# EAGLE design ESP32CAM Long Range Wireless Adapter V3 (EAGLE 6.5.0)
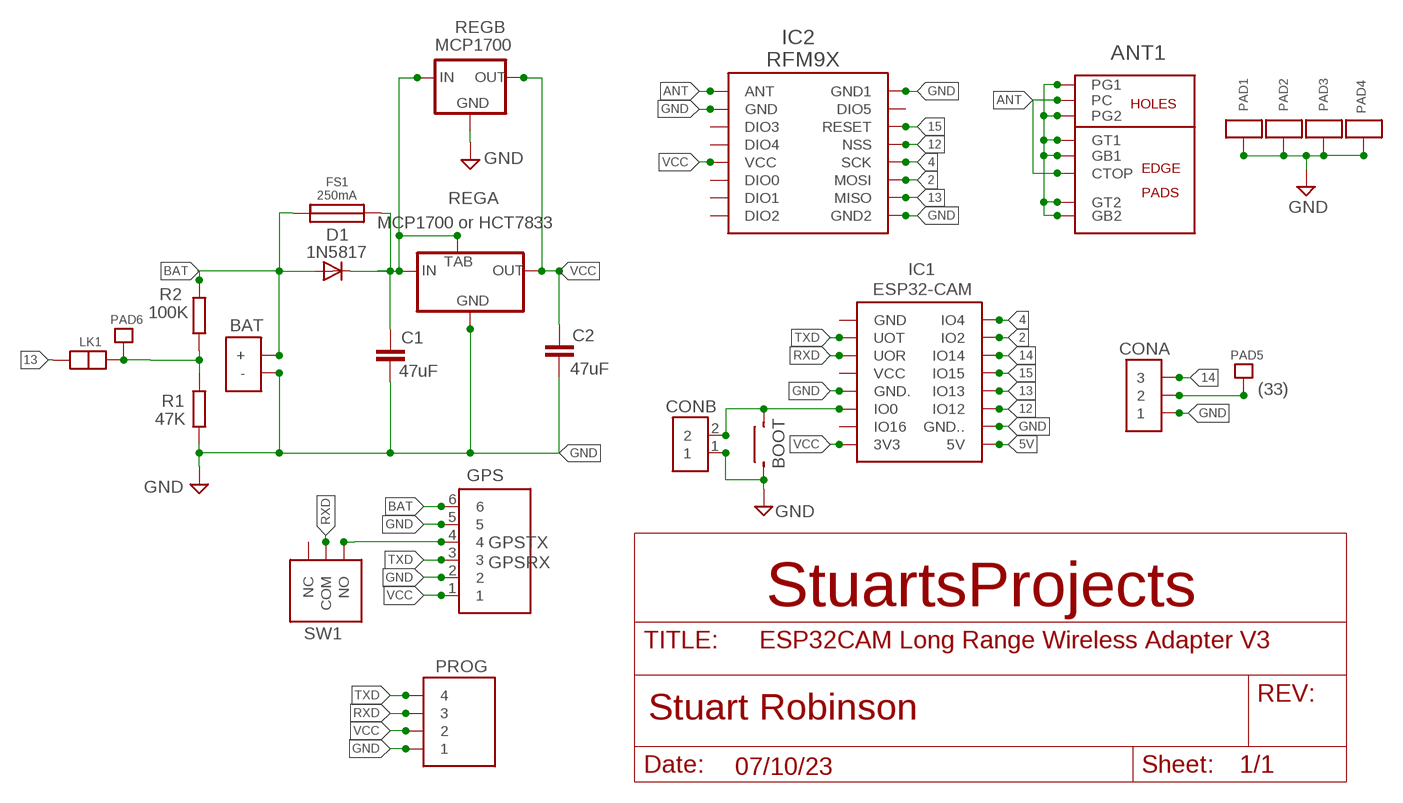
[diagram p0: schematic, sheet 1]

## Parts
ANT1  CUSTOMSMA  [CUSTOMSMA]
BAT  BATPADS2  [BATPADS]
BOOT  SMALLSMTSWITCH  [SMALLSMTSWITCH]
C1  47uF  C-EUC1206  [C1206]
C2  47uF  C-EUC1206  [C1206]
CONA  3X1  [3X1]
CONB  2X1  [2X1]
D1  1N5817  DIODE-DO41-7.6  [DO41-7.6]
FS1  250mA  SMALL_POLYFUSE  [SMALL_POLYFUSE]
GPS  6X1  [6X1]
IC1  ESP32-CAM  [ESP32-CAM]
IC2  RFM9X  RFM98_PIH  [RFM98_PIH]
LK1  2PADLINKLARGE  [2PADLINKLARGE]
PAD1  ANTPAD2  [ANTPAD2]
PAD2  ANTPAD2  [ANTPAD2]
PAD3  ANTPAD2  [ANTPAD2]
PAD4  ANTPAD2  [ANTPAD2]
PAD5  SINGLEPAD  [SINGLEPAD]
PAD6  SINGLEPAD  [SINGLEPAD]
PROG  4X1  [4X1]
R1  47K  125MWRESISTORSTANDARD  [125MWRESISTOR]
R2  100K  125MWRESISTORSTANDARD  [125MWRESISTOR]
REGA  MCP1700 or HCT7833  MCP1700SOT89  [MCP1700SOT89]
REGB  MCP1700  [TO92REGB]
SW1  SMALL_PCB_SLIDE_DEFAULT  [SMALL_PCB_SLIDE]

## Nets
2: IC1.IO2 IC2.MOSI
4: IC1.IO4 IC2.SCK
5V [POWER]: C1.1 D1.C FS1.P$2 IC1.5V REGA.2(IN) REGA.4(TAB) REGB.IN
12: IC1.IO12 IC2.NSS
13: IC1.IO13 IC2.MISO LK1.P$1
14: CONA.3 IC1.IO14
15: IC1.IO15 IC2.RESET
ANT: ANT1.CTOP ANT1.PC IC2.ANT
BAT [POWER]: BAT.BAT+(+) D1.A FS1.P$1 GPS.6 R2.P$1
GND [POWER]: ANT1.G1 ANT1.G2 ANT1.GB1 ANT1.GB2 ANT1.GT1 ANT1.GT2 BAT.BAT-V(-) BOOT.P$3 C1.2 C2.2 CONA.1 CONB.1 GPS.2 GPS.5 IC1.GND. IC1.GND.. IC2.GND IC2.GND1 IC2.GND2 PAD1.P$1 PAD2.P$1 PAD3.P$1 PAD4.P$1 PROG.1 R1.P$2 REGA.1(GND) REGB.GND
N$1: BOOT.P$4 CONB.2 IC1.IO0
N$2: CONA.2 PAD5.P$1
N$3: GPS.4 SW1.NO
PAD6: LK1.P$2 PAD6.P$1 R1.P$1 R2.P$2
RXD: IC1.UOR PROG.3 SW1.COM
TXD: GPS.3 IC1.UOT PROG.4
VCC [POWER]: C2.1 GPS.1 IC1.3V3 IC2.VCC PROG.2 REGA.3(OUT) REGB.OUT
Unconnected: IC1.GND IC1.IO16 IC1.VCC IC2.DIO0 IC2.DIO1 IC2.DIO2 IC2.DIO3 IC2.DIO4 IC2.DIO5 SW1.NC

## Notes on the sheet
- (33)
- GPSTX
- GPSRX
- StuartsProjects
- 07/10/23

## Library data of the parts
ANT1 = con-coax:CUSTOMSMA
BAT = LMA2:BATPADS2
BOOT = LMA2:SMALLSMTSWITCH
C1 C2 = resistor:C-EU: CAPACITOR, European symbol
CONA = My_Pin_Headers:3X1
CONB = My_Pin_Headers:2X1
D1 = diode:DIODE-: DIODE
FS1 = LMA2:SMALL_POLYFUSE
GPS = My_Pin_Headers:6X1
IC1 = esp32:ESP32-CAM
IC2 = LMA2:RFM98_PIH
LK1 = LMA2:2PADLINKLARGE
PAD1-PAD4 = LMA2:ANTPAD2
PAD5 PAD6 = LMA2:SINGLEPAD
PROG = My_Pin_Headers:4X1
R1 R2 = LMA2:125MWRESISTOR
REGA = LMA2:MCP1700SOT89
REGB = LMA2:MCP1700
SW1 = switch-tact:SMALL_PCB_SLIDE

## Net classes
0 default: width 0.254 mm
1 POWER: width 0.762 mm
2 VDD: width 0.762 mm
3 gpspower: width 0.762 mm

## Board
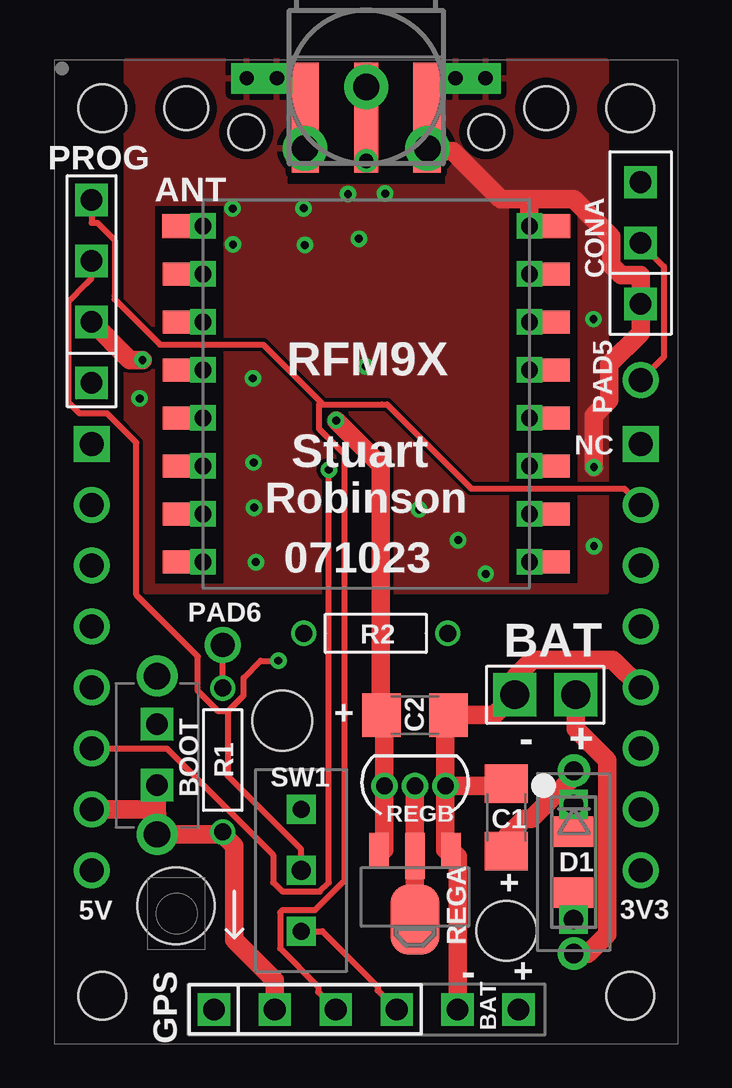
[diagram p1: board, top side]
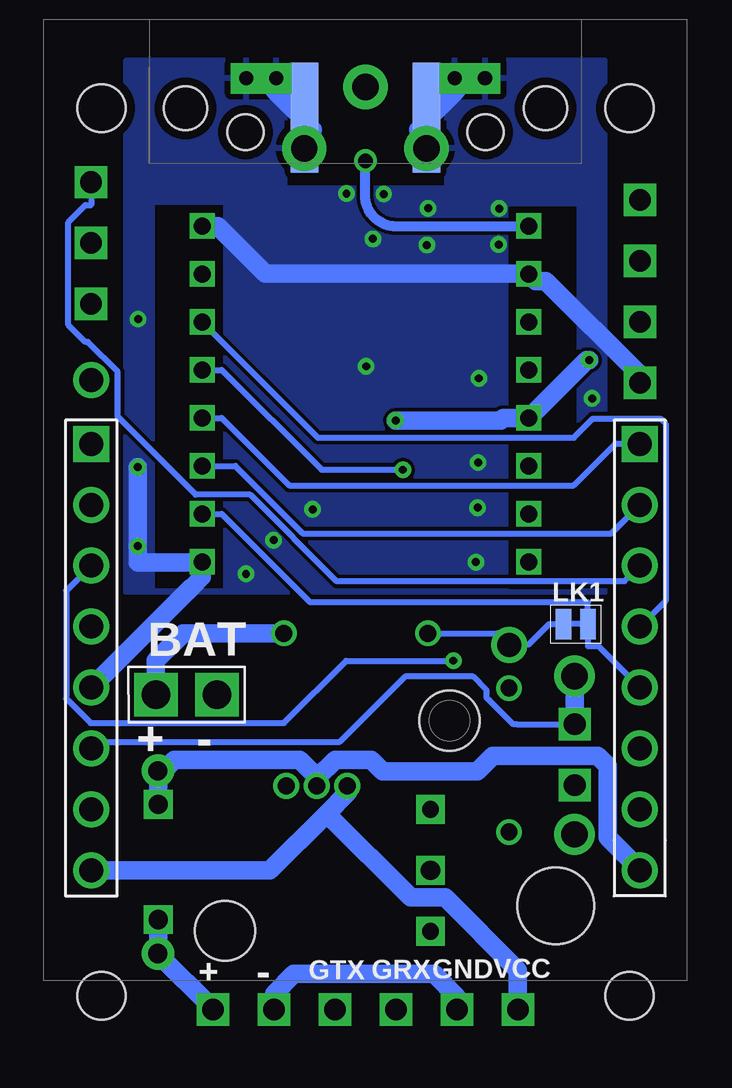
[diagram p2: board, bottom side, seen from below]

No outline drawn. Coordinates in mm, seen from the top.
Copper layers (1*16): Top 0.0356mm / dielectric 1.5011mm / Bottom 0.0356mm
Design rules "LaenPCBOrder *": minimum track width 6mil, minimum drill 13mil, track to track 6mil, track to pad 6mil, pad to pad 6mil, via to via 6mil, smd to smd 6mil, copper to edge 15mil, drill to drill 6mil, minimum pad ring 7mil, minimum via ring 7mil, stop-mask expansion 3mil, vias tented up to drill 1000mil, thermal gap 10mil
Holes 3.2 mm at 5.07,5.75
Holes 1.5 mm at 8,38 18,38
Holes 2.5 mm at 9.5,13.47 18.85,4.71
Holes 2 mm at 2,2 24,2 2,39 24,39
Holes 1.8 mm at 5.5,39 20.5,39
tRestrict: area 0,0 to 26.4,0.5; area 9.7,35.9 to 16.3,41; area 4.2,19.2 to 7,34.9; area 19,19.2 to 21.8,34.9
bRestrict: area 0,0 to 26.1,0.5; area 9.7,35.8 to 16.2,41; area 4.2,19 to 7,34.9; area 18.9,19 to 21.8,35

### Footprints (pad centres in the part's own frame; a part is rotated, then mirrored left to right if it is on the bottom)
CUSTOMSMA = smd 4.572 x 1.016: CTOP -1.27,0 | drill 1.1 pad 1.85: G1 -2.55,2.55; G2 -2.55,-2.55; PC 0,0 | smd 4.572 x 1.143 bottom: GB1 -1.27,2.54; GB2 -1.27,-2.54 | smd 4.572 x 1.143: GT1 -1.27,2.54; GT2 -1.27,-2.54
BATPADS = drill 1.2 pad 1.778 square: BAT+ 0,-1.27; BAT-V 0,1.27
SMALLSMTSWITCH = drill 1.1 pad 1.7: P$3 -3.3,0; P$4 3.3,0
C1206 = smd 1.6 x 1.8: 1 -1.4,0; 2 1.4,0
3X1 = drill 0.9 square: 1 -2.54,0; 2 0,0; 3 2.54,0
2X1 = drill 0.9 square: 1 -1.27,0; 2 1.27,0
DO41-7.6 = drill 0.8 pad 1.35: A 3.81,0; C -3.81,0
SMALL_POLYFUSE = drill 0.8 square: P$1 -2.4,0; P$2 2.4,0 | smd 1.27 x 1.635: P$3 -1.27,0; P$4 1.27,0
6X1 = drill 0.9 square: 1 -6.35,0; 2 -3.81,0; 3 -1.27,0; 4 1.27,0; 5 3.81,0; 6 6.35,0
ESP32-CAM = drill 1: 3V3 -11.43,3.81; 5V 11.43,3.81; GND. -11.43,11.43; GND.. 11.43,6.35; IO0 -11.43,8.89; IO2 11.43,19.05; IO12 11.43,8.89; IO13 11.43,11.43; IO14 11.43,16.51; IO15 11.43,13.97; IO16 -11.43,6.35; UOR -11.43,16.51; UOT -11.43,19.05; VCC -11.43,13.97 | drill 1 square: GND -11.43,21.59; IO4 11.43,21.59
RFM98_PIH = drill 0.7 pad 0.965 square: ANT -6.8,7.5; DIO0 -6.8,-2.5; DIO1 -6.8,-4.5; DIO2 -6.8,-6.5; DIO3 -6.8,3.5; DIO4 -6.8,1.5; DIO5 6.8,5.5; GND -6.8,5.5; GND2 6.8,-6.5; MISO 6.8,-4.5; MOSI 6.8,-2.5; NSS 6.8,1.5; RESET 6.8,3.5; SCK 6.8,-0.5; VCC -6.8,-0.5 | drill 0.7 pad 1.016 square: GND1 6.8,7.5 | smd 2.2 x 1: P$2 -7.4,7.5; P$6 7.4,7.5 | smd 2.159 x 0.965: P$4 -7.4,5.5; P$5 -7.4,1.5; P$7 7.4,5.5; P$9 -7.4,3.5; P$10 -7.4,-0.5; P$11 -7.4,-2.5; P$12 -7.4,-4.5; P$13 -7.4,-6.5; P$14 7.4,-6.5; P$15 7.4,-4.5; P$16 7.4,-2.5; P$17 7.4,-0.5; P$18 7.4,1.5; P$19 7.4,3.5
2PADLINKLARGE = smd 1.27 x 0.66: P$1 0,0.46; P$2 0,-0.56
ANTPAD2 = drill 0.6 pad 1.27 square: P$1 0,0
SINGLEPAD = drill 1: P$1 0,0
4X1 = drill 0.9 square: 1 -3.81,0; 2 -1.27,0; 3 1.27,0; 4 3.81,0
125MWRESISTOR = drill 0.7: P$1 -3,0; P$2 3,0
MCP1700SOT89 = smd 0.8 x 1.4: 1 -1.499,-1.981; 3 1.499,-1.981 | smd 0.8 x 1.9: 2 0,-1.727 | smd 2.032 x 2.921: 4 0,0.94
TO92REGB = drill 0.7 pad 1.1: GND -1.27,-1.2; IN 0,-1.2; OUT 1.27,-1.2
SMALL_PCB_SLIDE = drill 0.8 pad 1.2 square: COM 0,0 | drill 0.7 pad 1.2 square: NC 2.54,0; NO -2.54,0

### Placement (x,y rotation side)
ANT1  13,39.88 90 top
BAT  20.46,14.55 90 top
BOOT  4.29,12.03 90 top
C1  18.83,9.44 90 top
C2  15.03,13.7 0 top
CONA  24.43,33.38 90 top
CONB  4.28,12.05 90 top
D1  21.65,7.57 270 top
FS1  21.64,7.58 90 top
GPS  13,1.43 0 top
IC1  13,3.42 0 bottom
IC2  13,26.59 0 top
LK1  4.19,17.49 270 bottom
PAD1  16.72,40.25 0 top
PAD2  17.97,40.25 0 top
PAD3  8.02,40.25 0 top
PAD4  9.28,40.25 0 top
PAD5  24.43,27.66 0 top
PAD6  7.02,16.63 0 top
PROG  1.56,31.37 90 top
R1  7.02,11.83 270 top
R2  13.4,17.11 180 top
REGA  15.03,6.11 180 top
REGB  15.03,9.55 180 top
SW1  10.29,7.23 90 top

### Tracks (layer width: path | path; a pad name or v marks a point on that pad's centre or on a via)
2
  Bottom 0.254: IC2.MOSI 18.43,24.09 15.62,21.28 2.76,21.28 IC1.IO2
4
  Bottom 0.254: IC1.IO4 2.6,25.01 4.33,23.28 16.18,23.28 18.99,26.09 IC2.SCK
5V
  Top 0.762: D1.C 21.6,11.3 21.6,11.1 19.87,9.37 19.59,9.37 18.84,8.62 C1.1 | REGB.IN REGA.2 REGA.4
  Bottom 0.762: FS1.P$2 D1.C 21.3,11.5 20.96,11.84 15.74,11.84 15,11.1 | 15,11.1 REGB.IN | 15,11.1 14.26,11.84 12.77,11.84 12.29,11.36 8.34,11.36 7.7,12 3.33,12 2.9,11.57 2.9,8.6 1.6,7.3 IC1.5V
12  (via drill 0.33 pad 0.69)
  Top 0.254: IC1.IO12 4.7,12.31 9.12,7.88 9.12,6.73 9.5,6.35 11.07,6.35 11.44,6.72 v11.44,23.93 | v11.44,23.93
  Bottom 0.254: IC2.NSS 18.99,28.09 14.83,23.93 v11.44,23.93
13
  Bottom 0.254: IC2.MISO 18.99,22.09 15.31,18.4 3.73,18.4 LK1.P$1 3.73,16.58 3.3,16.58 IC1.IO13
14
  Bottom 0.254: CONA.3 24.43,34.97 24.67,34.97 25.38,34.25 25.38,29.97 24.67,29.25 24.57,29.25 23.33,28.01 23.33,26.15 20.07,22.9 17.81,22.9 14.19,19.28 2.22,19.28 IC1.IO14
15
  Bottom 0.254: IC2.RESET 14.98,25.27 4.32,25.27 3.53,26.06 0.7,26.06 0.49,25.85 0.49,18.46 IC1.IO15
ANT  (via drill 0.6 pad 0.69)
  Top 0.254: ANT1.CTOP ANT1.PC
  Top 0.406: v13,36.81 13.02,39.86 arc90 ANT1.PC
  Bottom 0.406: IC2.ANT 6.22,34.07 11.69,34.07 11.72,34.07 arc90 13.02,35.37 v13,36.81 | 13.02,39.86 arc90 ANT1.PC
BAT
  Top 0.762: BAT.BAT+ 21.73,13.12 23.03,11.81 23.03,4.56 22.24,3.76 D1.A
  Bottom 0.762: FS1.P$1 21.64,4.05 21.65,4.04 D1.A 19.35,1.46 GPS.6 | BAT.BAT+ 21.73,15.98 20.6,17.11 R2.P$1
GND  (via drill 0.33, 0.33 pad 0.69)
  Top 0.762: IC1.GND. 23.28,16 19.93,16 19.19,15.27 BAT.BAT-V 18.34,13.7 C2.2 16.3,13.7 REGB.GND | GPS.5 16.81,7.81 REGA.1 16.3,8.09 REGB.GND | 7.02,8.73 R1.P$2 | 7.02,8.73 7.5,8.25 7.5,4.33 9.19,2.64 GPS.2 | 7.02,8.73 BOOT.P$3 4.29,9.56 4.28,9.57 4.28,9.77 | ANT1.GT2 ANT1.G2 15.59,37.31 | 19.81,35.2 21.65,35.2 23.2,33.65 23.2,32.47 23.62,32.05 24.43,32.05 CONA.1 24.43,29.63 23.13,28.33 23.13,26.83 22.49,26.19 v22.49,24.04 | 15.59,37.31 15.9,37.2 16.6,37.2 18.6,35.2 19.81,35.2 | 15.59,37.31 | ANT1.G1 ANT1.GB1 | CONB.1 4.28,9.77 | IC1.GND.. 4.28,9.77 | 19.81,35.2 19.8,35.19 IC2.GND1 | REGB.GND 18.83,10.75 C1.2
  Bottom 0.762: 9.28,39.67 10.34,38.61 ANT1.GB1 10.46,37.46 10.52,37.4 ANT1.G1 10.8,38.1 | 16.72,39.67 15.66,38.61 ANT1.GT2 15.54,37.4 15.55,37.39 ANT1.G2 15.2,38.1 | PAD2.P$1 16.8,40.25 16.8,39.75 16.72,39.67 | PAD1.P$1 16.72,39.67 | PAD3.P$1 9.19,40.25 9.19,39.76 9.28,39.67 | PAD4.P$1 9.28,39.67 | IC1.GND. 20.25,19.03 20.24,19.03 19.82,19.45 19.82,20.07 | IC2.GND1 19.16,34.09 17.18,32.11 6.22,32.11 IC2.GND 5.91,31.8 5.49,31.8 1.56,27.87 PROG.1 | 19.82,20.07 IC2.GND2 | GPS.2 9.19,1.96 10.14,2.91 15.98,2.91 16.81,2.08 GPS.5 | 19.82,20.07 22.49,20.07 v22.49,20.75 v22.49,24.04
  other vias: 13.79,35.44 12.24,35.42 7.43,34.82 7.45,33.32 10.39,34.83 10.44,33.3 12.69,33.56 8.28,27.74 8.31,24.23 8.33,22.35 8.4,20.08 15.2,22.28 16.83,21 17.98,19.59 12.97,28.24 3.56,26.9 22.47,30.21
  pour Bottom: 3,41 23,41 23,18.83 3,18.83
  pour Top: 3,41 23,41 23,18.83 3,18.83
N$1
  Bottom 0.254: IC1.IO0 24.15,12.59 14.07,12.59 11.35,15.31 8.52,15.31 7.96,14.75 7.95,14.75 7.95,14.42 7.85,14.32 7.84,14.32 6.84,13.32 6.69,13.32 CONB.2
  Bottom 0.762: BOOT.P$4 CONB.2
N$2
  Top 0.254: CONA.2 24.5,33.3 25.4,32.4 25.4,28.63 PAD5.P$1
N$3
  Top 0.254: SW1.NO 11.17,4.69 13.47,2.38 13.47,2.23 GPS.4
N$4
  Bottom 0.254: 3.98,17.5 4.57,17.5 | 4.57,17.5 4.58,17.5 4.57,17.5
PAD6
  Top 0.254: R1.P$1 PAD6.P$1
  Bottom 0.254: R2.P$2 7.5,17.11 PAD6.P$1 6.22,16.63 5.36,17.49 LK1.P$2
RXD  (via drill 0.33 pad 0.69)
  Top 0.254: 7.23,13.86 7.23,11.17 10.29,8.11 SW1.COM | 7.23,13.86 6.84,13.86 5.99,14.71 5.99,16.14 3.42,18.71 3.42,25.06 2.44,26.04 2.2,26.28 1.05,26.28 0.61,26.73 0.61,30.97 1.32,31.69 1.56,31.92 PROG.3 | 7.23,13.86 7.89,14.52 7.89,15.26 8.59,15.96 v9.33,15.96 v9.34,15.97
  Bottom 0.254: IC1.UOR 25.48,18.89 25.48,14.39 24.45,13.37 16.4,13.37 13.8,15.97 v9.34,15.97
TXD
  Top 0.254: 11.2,26.65 11.03,26.65 11.03,25.64 12.09,24.58 12.09,6.8 10.86,5.57 9.5,5.57 9.41,5.48 9.41,3.97 11,2.38 11,2.16 GPS.3 | 11.2,26.65 13.66,26.65 13.87,26.65 17.38,23.14 23.76,23.14 IC1.UOT | PROG.4 1.56,34.23 1.8,34.23 2.51,33.51 2.51,31.18 2.51,31.04 4.41,29.14 8.71,29.14 11.2,26.65
VCC  (via drill 0.33 pad 0.69)
  Top 0.762: v11.74,25.98 13.61,24.12 13.61,15.13 C2.1 13.76,13.7 REGB.OUT 13.76,8.09 REGA.3 | PROG.2 3.15,28.51 v3.68,28.51
  Bottom 0.762: 14.62,9.59 16.98,7.23 IC1.3V3 | REGB.OUT 13.73,10.48 14.62,9.59 | 14.62,9.59 11.12,6.1 9.67,6.1 6.65,3.07 GPS.1 | v11.74,25.98 7.37,25.98 7.26,26.09 IC2.VCC 3.78,28.51 v3.68,28.51

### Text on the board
tPlace: ANT
tNames: PROG | CONA | RFM9X | PAD5 | NC | Stuart | Robinson | 071023 | PAD6 | R2 | BAT | BOOT | + | C2 | - | + | SW1 | R1 | REGB | C1 | + | D1 | 5V | 3V3 | REGA | - | + | GPS | BAT
bNames: LK1 | BAT | - | + | - | + | VCC | GND | GRX | GTX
